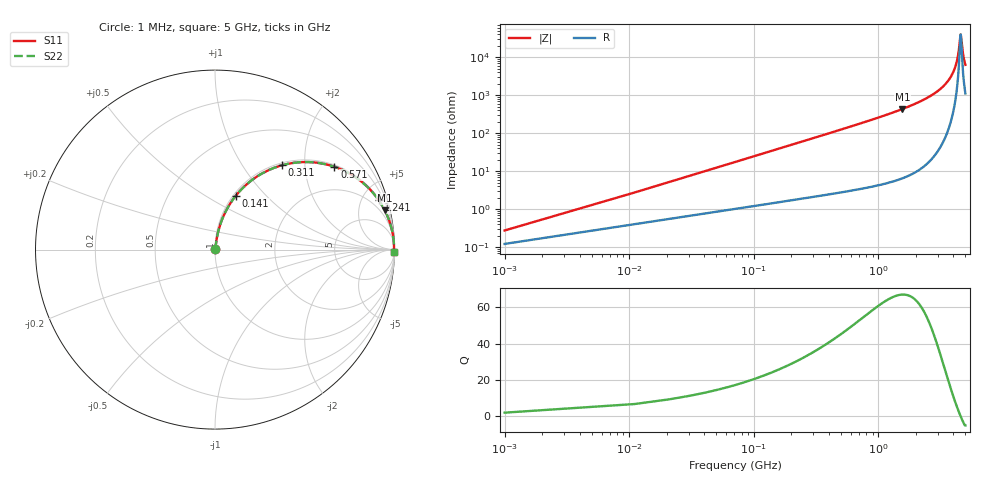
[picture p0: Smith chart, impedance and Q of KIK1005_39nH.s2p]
!version-3
!date-01.2023
!Series
# MHz S RI R 50
!Freq ReS11 ImS11 ReS21 ImS21 ReS12 ImS12 ReS22 ImS22
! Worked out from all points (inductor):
!   501 points, 1 MHz to 5 GHz, reference 50 ohm
!   read as one part in series: L = 39 nH near 21 MHz
!   highest Q = 66.9 at 1.561 GHz (marker M1), where L = 44.1 nH
!   self-resonance near 4.571 GHz
!   S11 on the Smith chart (normalised r, x): 1 MHz: 1.00, +0.00; 141 MHz: 1.03, +0.69; 311 MHz: 1.04, +1.53; 571 MHz: 1.06, +2.84; 1.241 GHz: 1.10, +6.56; 5 GHz: open
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1  0.00121 0.00244  0.9988 -0.00244  0.9988 -0.00244  0.00121 0.00244
31  0.0123 0.0745  0.9877 -0.0745  0.9877 -0.0745  0.0123 0.0745
41  0.0174 0.098  0.9826 -0.098  0.9826 -0.098  0.0174 0.098
81  0.0474 0.1871  0.9526 -0.1871  0.9526 -0.1871  0.0474 0.1871
141  0.1168 0.3012  0.8832 -0.3012  0.8832 -0.3012  0.1168 0.3012
211  0.2196 0.3974  0.7804 -0.3974  0.7804 -0.3974  0.2196 0.3974
311  0.3731 0.4699  0.6269 -0.4699  0.6269 -0.4699  0.3731 0.4699
571  0.6657 0.4614  0.3343 -0.4614  0.3343 -0.4614  0.6657 0.4614
841  0.8156 0.3792  0.1844 -0.3792  0.1844 -0.3792  0.8156 0.3792
1241  0.9115 0.2764  0.0885 -0.2764  0.0885 -0.2764  0.9115 0.2764
1561  0.9464 0.2179  0.0536 -0.2179  0.0536 -0.2179  0.9464 0.2179
1671  0.9544 0.2014  0.0456 -0.2014  0.0456 -0.2014  0.9544 0.2014
2501  0.985 0.1125  0.015 -0.1125  0.015 -0.1125  0.985 0.1125
3341  0.9947 0.0567  0.00526 -0.0567  0.00526 -0.0567  0.9947 0.0567
3831  0.9968 0.0318  0.00316 -0.0318  0.00316 -0.0318  0.9968 0.0318
4171  0.9974 0.0166  0.00256 -0.0166  0.00256 -0.0166  0.9974 0.0166
4371  0.9975 0.00831  0.00245 -0.00831  0.00245 -0.00831  0.9975 0.00831
4451  0.9975 0.00509  0.00246 -0.00509  0.00246 -0.00509  0.9975 0.00509
4551  0.9975 0.00115  0.00249 -0.00115  0.00249 -0.00115  0.9975 0.00115
4581  0.9975 -9.42e-06  0.00251 9.42e-06  0.00251 9.42e-06  0.9975 -9.42e-06
4791  0.9973 -0.00795  0.0027 0.00795  0.0027 0.00795  0.9973 -0.00795
5000  0.997 -0.0155  0.00302 0.0155  0.00302 0.0155  0.997 -0.0155
